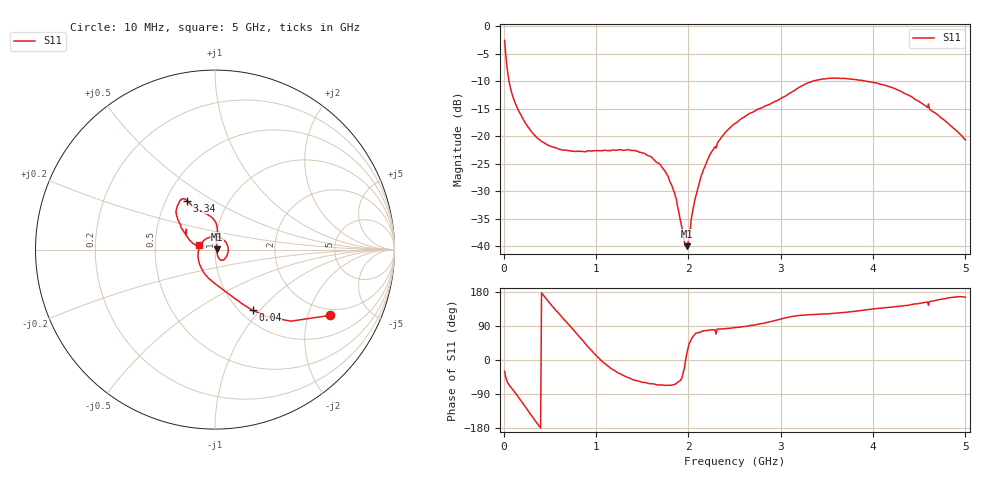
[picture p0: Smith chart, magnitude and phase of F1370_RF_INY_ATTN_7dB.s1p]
! S-parameters for RF_INY input IDT F1370 DPD Demodulator
! Date Measured:  2015-11-25  RGG
!  Port 1 = Pin 3 = RF_INY
! STATE: RF_INY selected, 7 dB attenuation (Gain = Gmax - 7 dB)
! RF Frequency:  10 MHz to 5000 MHz
! RF_INX, IF_I+, IF_I-, IF_Q+, and IF_Q- terminated
! 2300 MHz, 0 dBm signal applied to LO_IN
! Vcc = +5.00 Volts  Icc = approx 275 mA
! NOTES:  The device was measured on a custom printed circuit evaluation board with individual 50 ohm
!  microstrip lines to the RF and LO pins. The 50 ohm microstrip lines were de-embedded using reference
!  plane extensions
! Instrument Manufacturer:  Agilent Technologies
! Instrument Model:  E5071C
! Instrument Serial Number:  MY46419053
! Instrument Firmware Rev:  A.11.31
# HZ  S  RI R 50.00
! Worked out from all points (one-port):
!   500 points, 10 MHz to 5 GHz, reference 50 ohm
!   lowest |S11| = -40.0 dB at 1.98 GHz (marker M1), VSWR 1.02, Z = 51 + j0.217 ohm
!   |S11| at or under -10 dB: 57.87 MHz to 3.348 GHz (3.29 GHz wide, 193 % of centre); 3.915 GHz to end of sweep
!   S11 on the Smith chart (normalised r, x): 10 MHz: 1.73, -2.80; 40 MHz: 1.14, -0.91; 3.34 GHz: 0.64, +0.39; 5 GHz: 0.84, +0.04
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1e7  0.6432 -0.3663
4e7  0.2092 -0.3383
7e7  0.0979 -0.2633
1.1e8  0.0307 -0.213
2.5e8  -0.0789 -0.0976
4.1e8  -0.0894 0.00448
6.4e8  -0.0265 0.0698
9.5e8  0.0661 0.0315
1.26e9  0.0607 -0.0445
1.51e9  0.0359 -0.0604
1.69e9  0.0227 -0.0509
1.8e9  0.0152 -0.0354
1.85e9  0.013 -0.0277
1.89e9  0.0115 -0.0184
1.95e9  0.0106 -0.00542
1.98e9  0.00978 0.00213
2e9  0.0093 0.00627
2.08e9  0.00937 0.0268
2.18e9  0.0115 0.0518
2.34e9  0.013 0.0917
2.51e9  0.00961 0.1303
3.13e9  -0.1081 0.2305
3.34e9  -0.1562 0.2731
3.76e9  -0.1994 0.2623
4.13e9  -0.2154 0.1946
4.38e9  -0.1913 0.1381
4.59e9  -0.1624 0.0826
5e9  -0.0892 0.0234
